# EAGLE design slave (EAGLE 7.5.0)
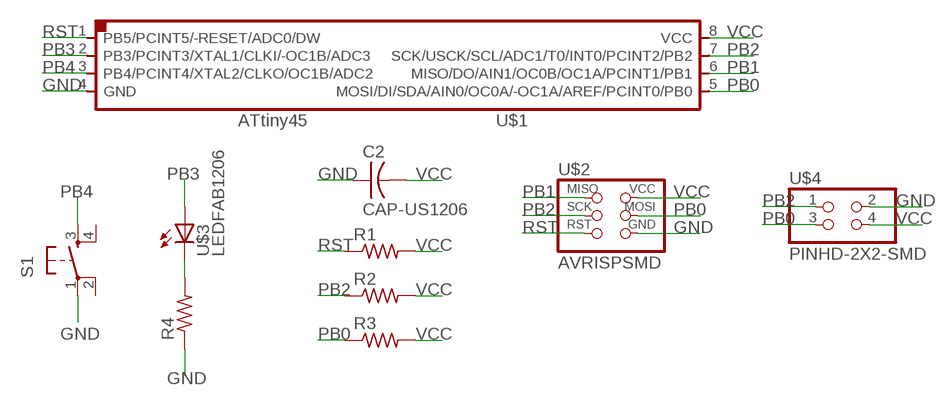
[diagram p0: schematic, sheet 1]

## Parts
C2  CAP-US1206  [C1206]
R1  RES-US1206  [R1206]
R2  RES-US1206  [R1206]
R3  RES-US1206  [R1206]
R4  RES-US1206  [R1206]
S1  6MM_SWITCH6MM_SWITCH  [6MM_SWITCH]
U$1  ATTINY45SI  [SOIC8]
U$2  AVRISPSMD  [2X03SMD]
U$3  LEDFAB1206  [LED1206FAB]
U$4  PINHD-2X2-SMD  [2X02SMD]

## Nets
GND: C2.1 R4.1 S1.1(P) U$1.4(GND) U$2.6(GND) U$4.2
N$2: R4.2 U$3.2(C)
PB0: R3.1 U$1.5(MOSI/DI/SDA/AIN0/OC0A/-OC1A/AREF/PCINT0/PB0) U$2.4(MOSI) U$4.3
PB1: U$1.6(MISO/DO/AIN1/OC0B/OC1A/PCINT1/PB1) U$2.1(MISO)
PB2: R2.1 U$1.7(SCK/USCK/SCL/ADC1/T0/INT0/PCINT2/PB2) U$2.3(SCK) U$4.1
PB3: U$1.2(PB3/PCINT3/XTAL1/CLKI/-OC1B/ADC3) U$3.1(A)
PB4: S1.3(S) U$1.3(PB4/PCINT4/XTAL2/CLKO/OC1B/ADC2)
RST: R1.1 U$1.1(PB5/PCINT5/-RESET/ADC0/DW) U$2.5(RST)
VCC: C2.2 R1.2 R2.2 R3.2 U$1.8(VCC) U$2.2(VCC) U$4.4
Unconnected: S1.2(P1) S1.4(S1)

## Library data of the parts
C2 = fab:CAP-US
R1-R4 = fab:RES-US: Resistor (US Symbol)
S1 = fab:6MM_SWITCH: OMRON SWITCH
U$1 = fab:ATTINY45
U$2 = fab:AVRISP
U$3 = fab:LED: LED
U$4 = fab:PINHD-2X2-SMD

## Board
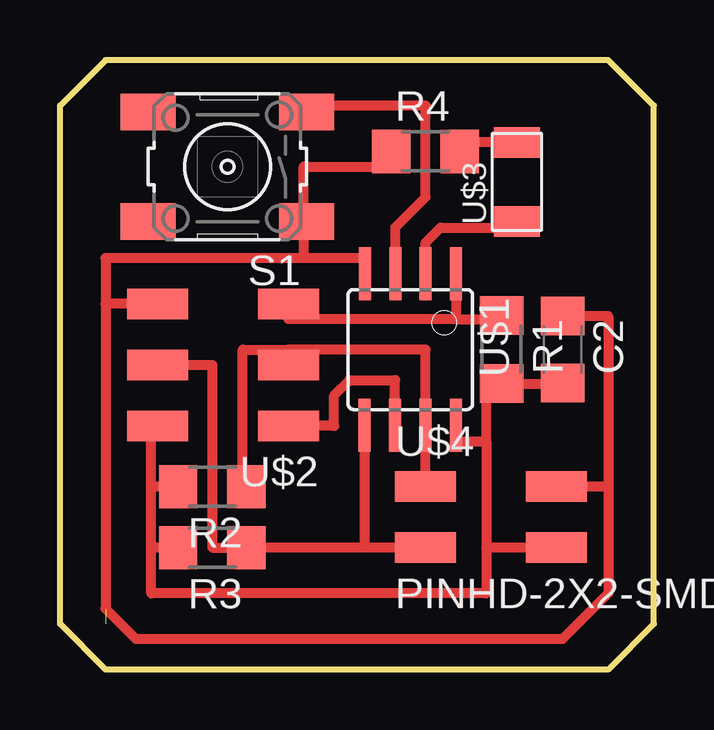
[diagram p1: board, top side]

Size 24.76 x 25.4 mm. Coordinates in mm from the lower left corner, seen from the top.
Outline: 22.86,0 1.9,0 0,1.91 0,23.5 1.9,25.4 22.86,25.4 24.76,23.5 24.76,1.91 22.86,0
Copper layers (1*16): Top 0.035mm / dielectric 1.5mm / Bottom 0.035mm
Design rules "default": minimum track width 10mil, minimum drill 24mil, track to track 8mil, track to pad 8mil, pad to pad 8mil, via to via 8mil, smd to smd 8mil, copper to edge 40mil, drill to drill 8mil, minimum pad ring 10mil, minimum via ring 8mil, stop-mask expansion 4mil, vias tented up to drill 0mil, thermal gap 10mil

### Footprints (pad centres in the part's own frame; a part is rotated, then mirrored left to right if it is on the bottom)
C1206 = smd 1.6 x 1.8: 1 -1.4,0; 2 1.4,0
R1206 = smd 1.6 x 1.803: 1 -1.422,0; 2 1.422,0
6MM_SWITCH = smd 2.286 x 1.524: 1 -3.302,2.286; 2 3.302,2.286; 3 -3.302,-2.286; 4 3.302,-2.286
SOIC8 = smd 0.5 x 2.2: 1 -1.905,-3.154; 2 -0.645,-3.154; 3 0.625,-3.154; 4 1.895,-3.154; 5 1.905,3.154; 6 0.635,3.154; 7 -0.635,3.154; 8 -1.905,3.154
2X03SMD = smd 2.54 x 1.27: 1 -2.54,2.54; 2 2.92,2.54; 3 -2.54,0; 4 2.92,0; 5 -2.54,-2.54; 6 2.92,-2.54
LED1206FAB = smd 1.27 x 1.905: 1 -1.651,0; 2 1.651,0
2X02SMD = smd 2.54 x 1.27: 1 -2.54,1.27; 2 2.92,1.27; 3 -2.54,-1.27; 4 2.92,-1.27

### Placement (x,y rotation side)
C2  20.95,13.34 270 top
R1  18.41,13.34 270 top
R2  6.35,7.62 180 top
R3  6.35,5.08 180 top
R4  15.24,21.59 0 top
S1  6.98,20.95 180 top
U$1  14.6,13.34 180 top
U$2  6.98,12.7 180 top
U$3  19.05,20.32 90 top
U$4  17.78,6.35 0 top

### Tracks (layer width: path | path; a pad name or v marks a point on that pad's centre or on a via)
GND  (1 unrouted)
  Top 0.406: U$1.4 12.7,16.49 12.7,17.15 10.16,17.15 | 10.16,17.15 1.9,17.15 1.9,15.24 | 1.9,15.24 1.9,2.54 3.17,1.27 20.95,1.27 22.86,3.18 22.86,7.62 | 22.86,7.62 U$4.2 | C2.1 22.86,14.73 22.86,7.62 | 10.16,18.67 10.16,17.15 | S1.1 10.16,18.67 | 10.16,18.67 10.16,20.95 13.82,20.95 | 13.97,20.95 13.82,20.95 | 13.82,20.95 R4.1 | U$2.6 1.9,15.24
N$2
  Top 0.406: U$3.2 16.66,21.97 R4.2
PB0
  Top 0.406: U$4.3 12.7,5.08 | U$2.4 6.35,12.7 6.35,5.08 R3.1 12.7,5.08 | U$1.5 12.7,5.08
PB1
  Top 0.406: U$1.6 13.97,12.07 12.06,12.07 11.43,11.43 11.43,10.16 U$2.1
PB2
  Top 0.406: 9.52,13.34 15.24,13.34 U$1.7 U$4.1 | 9.52,13.34 U$2.3 | R2.1 7.62,7.62 7.62,13.34 9.52,13.34
PB3
  Top 0.406: U$1.2 15.24,17.78 15.87,18.41 18.8,18.41 U$3.1 19.05,18.41
PB4
  Top 0.406: S1.3 10.29,23.5 15.24,23.5 15.24,19.69 13.98,18.43 U$1.3
RST
  Top 0.406: U$1.1 16.51,14.61 | 16.51,14.61 18.41,14.61 R1.1 | 16.51,14.61 9.52,14.61 U$2.5
VCC
  Top 0.406: C2.2 20.95,11.91 R1.2 18.41,12.07 17.78,12.07 17.78,9.53 | U$1.8 16.51,9.53 17.78,9.53 | 17.78,9.53 17.78,5.08 | U$4.4 17.78,5.08 | 17.78,5.08 17.78,3.18 3.81,3.18 3.81,5.08 | 3.81,5.08 3.81,7.62 | 3.81,7.62 3.81,10.16 U$2.2 | R3.2 3.81,5.08 | R2.2 3.81,7.62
